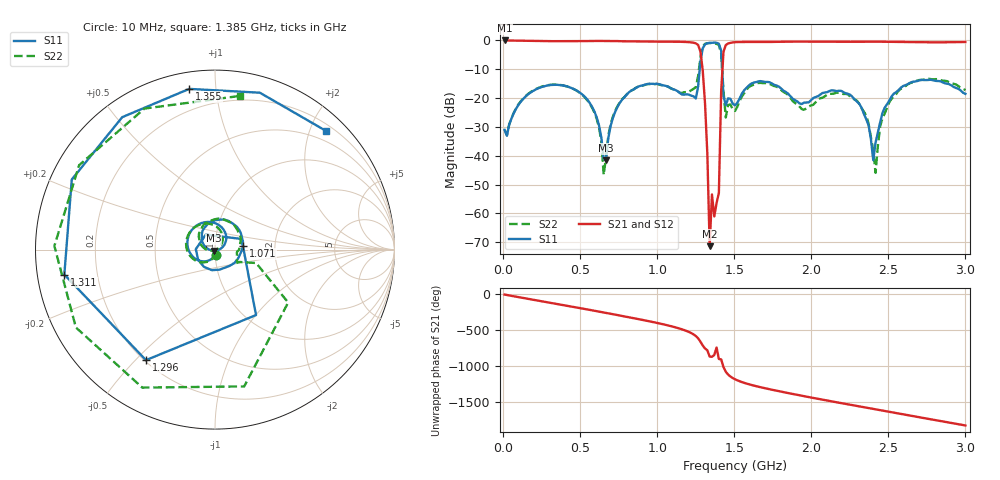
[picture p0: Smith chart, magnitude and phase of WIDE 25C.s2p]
!Agilent Technologies,E8363B,SG43030131,A.07.50.48
!Agilent E8363B: A.07.50.48
!Date: Friday, November 21, 2025 21:47:02
!Correction: S11(Full 2 Port(1,2))
!S21(Full 2 Port(1,2))
!S12(Full 2 Port(1,2))
!S22(Full 2 Port(1,2))
!S2P File: Measurements: S11, S21, S12, S22:
# Hz S  dB  R 50
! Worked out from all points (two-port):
!   201 points, 10 MHz to 3 GHz, reference 50 ohm
!   highest |S21| = -0.06 dB at 10 MHz (marker M1); lowest = -71.3 dB at 1.341 GHz (marker M2)
!   |S21| within 3 dB of the highest: start of sweep to 1.275 GHz; 1.436 GHz to end of sweep
!   lowest |S11| = -41.6 dB at 667.8 MHz (marker M3), VSWR 1.02, Z = 49.4 - j0.578 ohm
!   |S11| at or under -10 dB: start of sweep to 1.276 GHz; 1.421 GHz to end of sweep
!   |S22| runs from -46.6 to -1.0 dB; largest |S21 - S12| = 0.023
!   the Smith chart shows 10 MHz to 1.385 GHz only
!   S11 on the Smith chart (normalised r, x): 10 MHz: 1.01, -0.06; 1.071 GHz: 1.37, +0.06; 1.296 GHz: 0.21, -0.54; 1.311 GHz: 0.08, -0.08; 1.355 GHz: 0.08, +0.85; 1.385 GHz: 0.31, +2.27
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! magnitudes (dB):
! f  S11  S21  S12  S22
! 10 MHz  -31.1  -0.1  0.0  -31.0
! 219.3 MHz  -16.9  -0.2  -0.2  -16.7
! 518.3 MHz  -19.0  -0.3  -0.3  -19.1
! 667.8 MHz  -41.6  -0.2  -0.2  -40.6
! 757.5 MHz  -21.7  -0.3  -0.3  -21.5
! 1.012 GHz  -15.2  -0.5  -0.5  -15.3
! 1.071 GHz  -16.1  -0.5  -0.5  -16.1
! 1.251 GHz  -20.2  -1.1  -1.1  -16.3
! 1.296 GHz  -2.8  -10.5  -10.5  -2.2
! 1.311 GHz  -1.4  -22.0  -22.0  -1.2
! 1.341 GHz  -0.9  -71.3  -71.7  -1.0
! 1.355 GHz  -0.8  -53.4  -53.4  -1.0
! 1.385 GHz  -0.9  -56.4  -56.4  -1.2
! 1.4 GHz  -1.2  -52.9  -52.9  -1.7
! 1.415 GHz  -3.6  -17.6  -16.5  -4.7
! 1.43 GHz  -19.4  -4.0  -4.0  -17.5
! 1.505 GHz  -22.6  -0.7  -0.7  -24.5
! 2.013 GHz  -20.0  -0.5  -0.5  -22.3
! 2.297 GHz  -21.3  -0.5  -0.5  -21.0
! 2.417 GHz  -35.5  -0.5  -0.5  -45.9
! 2.507 GHz  -20.9  -0.5  -0.5  -21.4
! 3 GHz  -18.6  -0.6  -0.6  -17.3
